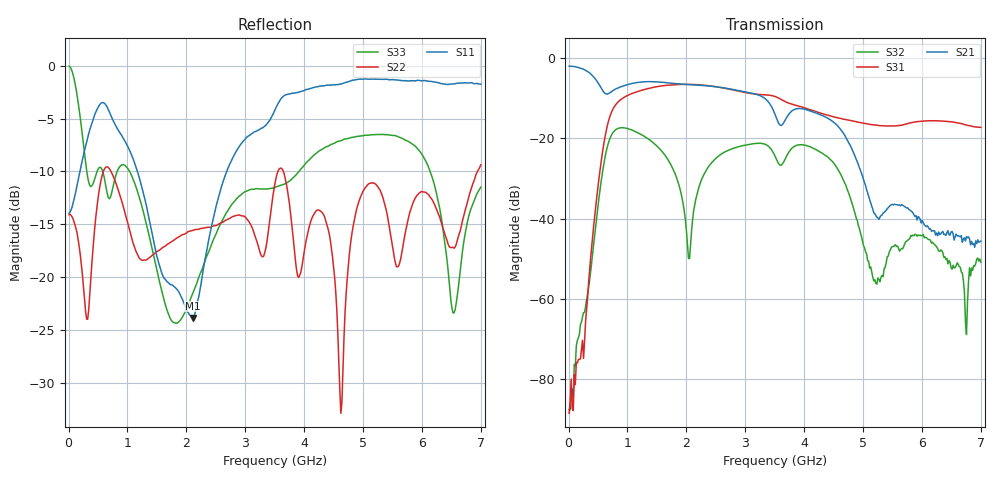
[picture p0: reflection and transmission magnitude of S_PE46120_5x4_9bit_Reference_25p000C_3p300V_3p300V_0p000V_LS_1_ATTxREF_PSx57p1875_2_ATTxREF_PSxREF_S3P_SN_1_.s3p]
! Device ID: PE46120_5x4_9bit_Reference
! Device ID: PE46120_5x4_9bit_Reference
! File Path: z:\PE46120_5x4_9bit_Reference\MPAC_Yi\new_12port\25p000C\3p300\LS_1_ATTxREF_PSx57p1875_2_ATTxREF_PSxREF\PE46120_5x4_9bit_Reference_25p000C_3p300V_3p300V_0p000V_LS_1_ATTxREF_PSx57p1875_2_ATTxREF_PSxREF_S3P_SN_1_.s3p
! Serial: 1
! Lot:
! Temp: 25.000C
! VDD: 3.300
! VSS: 0.000
! Control_Hi: 3.300
! Control_Lo: 0.000
! Logic State: LS_1_ATTxREF_PSx57p1875_2_ATTxREF_PSxREF
! Port 1: RFin
! Port 2: RFout1
! Port 3: RFout2
! ThroughPath:1-2
! IDD: -0.0005397672
! ISS: 0
! Comment:
#  Hz  S  RI  R  50
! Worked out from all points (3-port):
!   401 points, 10 MHz to 7 GHz, reference 50 ohm
!   strongest paths, dB at 10 MHz, 1.758 GHz, 3.505 GHz, 5.253 GHz, 7 GHz:
!     S21: -1.9, -6.2, -14.0, -39.8, -45.6
!     S31: -88.6, -6.6, -9.5, -16.7, -17.2
!     S32: -87.7, -27.1, -24.4, -54.8, -50.9
!   lowest |S11| = -23.8 dB at 2.107 GHz (marker M1), VSWR 1.14, Z = 53.9 + j5.44 ohm
!   |S11| at or under -10 dB: start of sweep to 193.2 MHz; 1.169 GHz to 2.685 GHz (1.516 GHz wide, 78.7 % of centre)
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1e7  0.1999 -0.0163  0.7895 -0.03  -7.27e-05 -5.76e-05
     0.7986 -0.0304  0.1976 -0.00597  2.34e-05 7e-06
     -2.1e-06 -3.71e-05  -3.69e-05 -1.85e-05  0.9883 -0.0962
2.5465e8  -0.00381 -0.3796  0.4201 -0.586  -0.000137 7.66e-05
          0.4261 -0.5942  0.081 -0.0394  -3.38e-05 0.000623
          -0.000165 7.23e-05  -7.68e-05 0.000667  -0.3295 -0.2636
7.61425e8  -0.5173 0.1775  -0.1552 -0.3624  -0.2333 -0.0334
           -0.157 -0.3673  0.2368 -0.1827  -0.0174 0.1179
           -0.236 -0.0336  -0.0174 0.1191  0.2483 -0.1107
1.390525e9  -0.0521 0.168  -0.4501 0.2317  0.4132 -0.088
            -0.4551 0.2352  0.0537 -0.1129  -0.0926 -0.0132
            0.4172 -0.0895  -0.0935 -0.0131  -0.1422 -0.0416
2.107e9  0.0401 0.0503  0.3573 0.2925  -0.3981 -0.2433
         0.3622 0.2955  -0.0679 -0.1522  -0.00835 0.00534
         -0.4032 -0.2456  -0.00823 0.0054  -0.0817 0.0196
3.505e9  -0.4456 -0.4282  -0.1651 0.1085  0.3279 0.0413
         -0.1672 0.1102  0.1056 0.2575  -0.0573 0.0162
         0.3319 0.0412  -0.0581 0.0165  0.192 -0.1848
4.6234e9  -0.8169 0.0494  0.0843 -0.0944  -0.0717 -0.1597
          0.0855 -0.0963  -0.0159 -0.0164  0.0066 -0.0344
          -0.0729 -0.162  0.00647 -0.0348  -0.2699 0.3495
5.200075e9  -0.7795 0.3672  -0.00574 -0.0097  -0.1406 -0.0366
            -0.00557 -0.0101  0.1674 -0.221  -0.000527 0.0011
            -0.1428 -0.0363  -0.000623 0.0016  0.2036 0.4256
6.528175e9  -0.2932 0.7642  0.00515 0.00358  0.0651 0.144
            0.00542 0.00357  -0.1386 -0.00595  0.00228 0.00149
            0.0665 0.1458  0.00232 0.00121  0.0679 0.00314
7e9  -0.1168 0.8072  0.00363 -0.00269  0.123 0.056
     0.00396 -0.00345  0.1033 0.3242  0.00171 0.0021
     0.1257 0.0561  0.00106 0.00265  0.1468 0.2228
